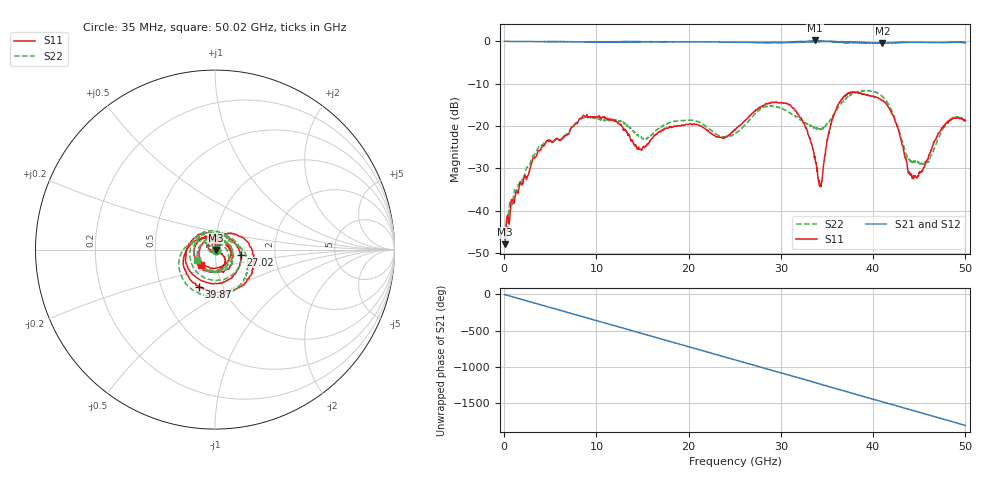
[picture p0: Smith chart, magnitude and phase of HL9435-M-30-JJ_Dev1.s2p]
! 5/26/2020 3:45:58 PM
! H:\PRODUCTION_DATA\TEMP_S2P.S2P
! CHANNEL.1
! TR.MEASUREMENT
! CORRECTED.DATA
# GHZ S RI R 50.0
! FREQ.GHZ  S11RE  S11IM  S21RE  S21IM  S12RE  S12IM  S22RE  S22IM
!; PortSelection: Port_12
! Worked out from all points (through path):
!   1429 points, 35 MHz to 50.02 GHz, reference 50 ohm
!   highest |S21| = 0.16 dB at 33.7 GHz (marker M1); lowest = -0.5 dB at 41.02 GHz (marker M2)
!   group delay of S21, straight-line fit = 101 ps
!   lowest |S11| = -47.8 dB at 35 MHz (marker M3), VSWR 1.01, Z = 50.4 - j0.188 ohm
!   |S11| at or under -10 dB: start of sweep to end of sweep
!   |S22| runs from -48.3 to -11.6 dB; largest |S21 - S12| = 0.048
!   S11 on the Smith chart (normalised r, x): 35 MHz: 1.01, -0.00; 27.02 GHz: 1.33, -0.08; 39.87 GHz: 0.77, -0.34; 50.02 GHz: 0.85, -0.15
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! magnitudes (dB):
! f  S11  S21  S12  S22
! 35 MHz  -47.8  0.0  0.0  -48.3
! 805 MHz  -37.3  -0.1  -0.1  -38.4
! 3.675 GHz  -25.9  -0.1  -0.1  -25.2
! 8.365 GHz  -18.2  -0.2  -0.2  -18.3
! 12.07 GHz  -18.9  -0.2  -0.2  -18.6
! 14.66 GHz  -25.4  -0.1  -0.2  -22.5
! 16.7 GHz  -21.6  -0.2  -0.1  -20.7
! 25.02 GHz  -20.8  -0.2  -0.3  -21.8
! 27.02 GHz  -16.8  -0.4  -0.2  -17.5
! 30.87 GHz  -14.9  -0.2  -0.2  -16.7
! 33.39 GHz  -24.8  -0.1  0.0  -20.0
! 33.7 GHz  -27.4  0.2  -0.1  -20.4
! 34.34 GHz  -34.3  -0.1  -0.1  -20.9
! 35.38 GHz  -19.9  -0.1  -0.1  -18.6
! 36.78 GHz  -13.2  -0.1  -0.3  -14.2
! 39.87 GHz  -12.9  -0.4  -0.5  -11.8
! 41.02 GHz  -14.0  -0.5  -0.5  -13.1
! 41.69 GHz  -15.6  -0.4  -0.4  -14.9
! 44.45 GHz  -31.9  -0.3  -0.3  -28.1
! 45.92 GHz  -27.8  -0.3  -0.3  -28.5
! 47.7 GHz  -19.8  -0.3  -0.3  -20.3
! 50.02 GHz  -18.7  -0.4  -0.3  -18.7
